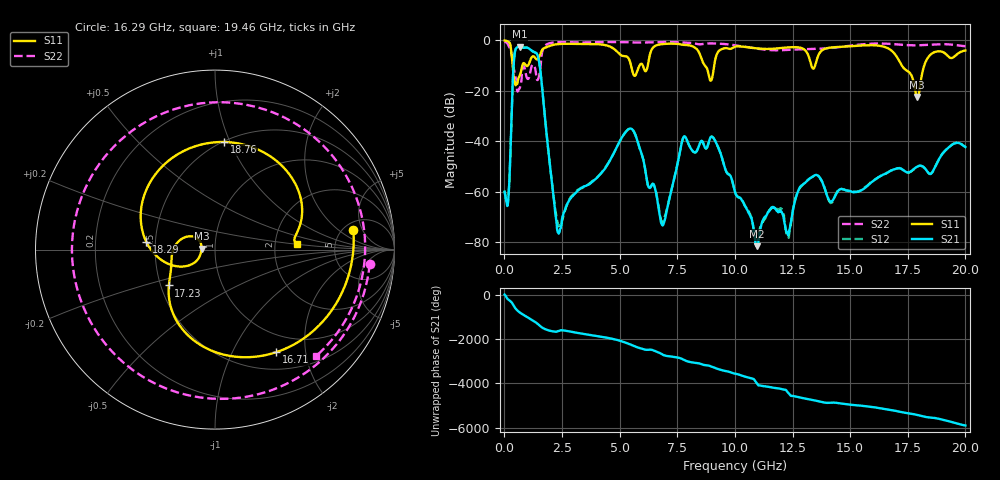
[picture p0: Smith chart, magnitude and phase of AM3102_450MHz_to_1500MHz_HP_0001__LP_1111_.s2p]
!Agilent Technologies,E8364B,MY43040894,A.07.50.67
!Agilent E8364B: A.07.50.67
!Date: Thursday, January 11, 2018 05:23:15
!Correction: S11(Full 2 Port(1,2))
!S21(Full 2 Port(1,2))
!S12(Full 2 Port(1,2))
!S22(Full 2 Port(1,2))
!S2P File: Measurements: S11, S21, S12, S22:
# Hz S  dB  R 50
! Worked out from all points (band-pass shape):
!   1601 points, 10 MHz to 20 GHz, reference 50 ohm
!   highest |S21| = -2.56 dB at 659.7 MHz (marker M1); lowest = -81.6 dB at 10.95 GHz (marker M2)
!   |S21| within 3 dB of the highest: 441.6 MHz to 1.422 GHz (980.8 MHz wide, 105 % of centre)
!   lowest |S11| = -22.5 dB at 17.91 GHz (marker M3), VSWR 1.16, Z = 43 + j0.413 ohm
!   |S11| at or under -10 dB: 359 MHz to 777.5 MHz (418.5 MHz wide, 73.7 % of centre); 8.701 GHz to 9.101 GHz (399.7 MHz wide, 4.49 % of centre); 17.24 GHz to 18.21 GHz (970.3 MHz wide, 5.47 % of centre)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
!   |S22| runs from -20.3 to -0.5 dB; largest |S21 - S12| = 0.0021
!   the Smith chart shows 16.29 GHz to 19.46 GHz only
!   S11 on the Smith chart (normalised r, x): 16.29 GHz: 6.05, +3.43; 16.71 GHz: 0.73, -1.50; 17.23 GHz: 0.55, -0.25; 18.29 GHz: 0.44, +0.05; 18.76 GHz: 0.51, +0.95; 19.46 GHz: 2.66, +0.19
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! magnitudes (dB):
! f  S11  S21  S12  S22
! 10 MHz  0.0  -60.0  -59.6  -0.5
! 184.9 MHz  -0.6  -61.2  -61.0  -2.2
! 447.3 MHz  -16.7  -5.1  -5.1  -13.0
! 659.7 MHz  -14.1  -2.6  -2.6  -19.0
! 1.484 GHz  -7.0  -7.4  -7.4  -14.9
! 2.334 GHz  -1.5  -76.3  -73.3  -0.7
! 3.346 GHz  -1.4  -58.4  -58.6  -0.8
! 5.482 GHz  -9.5  -35.0  -35.0  -0.8
! 6.682 GHz  -1.7  -65.9  -65.5  -0.7
! 7.819 GHz  -1.8  -38.1  -38.1  -0.9
! 10.01 GHz  -2.6  -60.1  -60.1  -2.0
! 10.95 GHz  -3.2  -81.6  -79.0  -3.3
! 13.34 GHz  -10.6  -54.2  -54.2  -3.5
! 16.29 GHz  -2.2  -54.0  -54.0  -1.3
! 16.68 GHz  -3.3  -52.2  -52.1  -1.4
! 16.71 GHz  -3.5  -52.0  -51.9  -1.4
! 17.23 GHz  -9.7  -51.0  -50.9  -1.7
! 17.91 GHz  -22.5  -50.1  -50.0  -2.0
! 18.29 GHz  -8.3  -51.3  -51.4  -1.8
! 18.76 GHz  -4.4  -48.7  -48.7  -1.6
! 19.46 GHz  -6.8  -41.2  -41.1  -1.7
! 20 GHz  -4.0  -42.3  -42.3  -2.3
